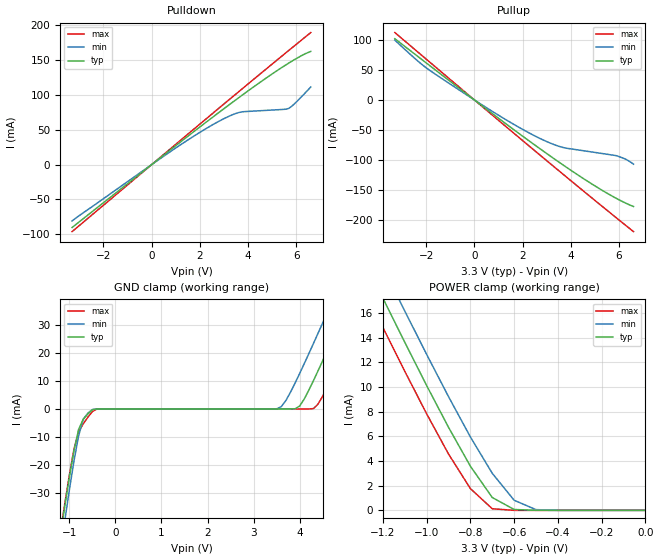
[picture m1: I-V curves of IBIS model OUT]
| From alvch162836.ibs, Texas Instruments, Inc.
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|   Model ALVCH162836_OUT
[Model]   OUT
Model_type   3-state
Polarity   Non-Inverting
Enable   Active-High
|Variable   typ   min   max
C_comp   7.0pF   NA   NA
[Voltage range]   3.3   3.0   3.6
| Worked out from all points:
|   slope of the pulldown table from 0 to 0.495 V, typ, clamps not added: 36.6 ohm
|   slope of the pullup table from 0 to 0.495 V, typ, clamps not added: 32.7 ohm
|   GND clamp passes 1 mA (typ) near -0.55 V on its own axis
|   POWER clamp passes 1 mA (typ) near -0.70 V on its own axis
[Pullup]   | Note: Vtable = Vcc - Voutput
|   Voltage   I(typ)   I(min)   I(max)
-3.3V     101.7mA    99.31mA    111.9mA
-2.3V     70.82mA    63.05mA    78mA
-1.8V     55.39mA    47.67mA    61.05mA
700mV     -21.34mA   -17.91mA   -23.7mA
2.4V      -71.8mA    -57.51mA   -80.85mA
3.1V      -91.84mA   -70.88mA   -104.2mA
3.6V      -105.8mA   -78.13mA   -120.8mA
4.9V      -140.3mA   -86.6mA    -163.6mA
5.9V      -163.8mA   -92.71mA   -196.2mA
6.3V      -171.8mA   -98.96mA   -209.1mA
6.6V      -177mA     -106.6mA   -218.7mA
[Pulldown]
|   Voltage   I(typ)   I(min)   I(max)
-3.3V     -90.25mA   -80.85mA   -96.21mA
700mV     19.09mA    16.83mA    20.42mA
1.7V      46.04mA    39.78mA    49.49mA
2.6V      69.89mA    58.61mA    75.55mA
3.2V      85.5mA     69.31mA    92.86mA
3.7V      98.3mA     75.47mA    107.2mA
5.5V      141.7mA    79.34mA    158.6mA
5.7V      146mA      80.98mA    164.3mA
6V        152.3mA    89.88mA    172.7mA
6.6V      162.5mA    111.4mA    189.6mA
[POWER_Clamp]   | Note: Vtable = Vcc - Voutput
|   Voltage   I(typ)   I(min)   I(max)
-3.3V     95.82mA    98.2mA     93.52mA
-1.3V     20.85mA    23.37mA    18.46mA
-1.2V     17.22mA    19.76mA    14.85mA
-1.1V     13.64mA    16.18mA    11.29mA
-1V       10.13mA    12.66mA    7.835mA
-900mV    6.739mA    9.228mA    4.573mA
-800mV    3.582mA    5.956mA    1.766mA
-700mV    1.041mA    3.004mA    129uA
-600mV    70.56uA    819.7uA    1.512uA
-500mV    2.077uA    58.75uA    22.94nA
0V        990pA      903.2pA    1.08nA
[GND_Clamp]
|   Voltage   I(typ)   I(min)   I(max)
-3.3V     -303.1mA   -308.7mA   -297.8mA
-1.2V     -45.81mA   -51.34mA   -44.52mA
-1.1V     -34.74mA   -39.9mA    -33.79mA
-800mV    -7.335mA   -9.635mA   -8.16mA
-400mV    -9.992nA   -367.3nA   -984.6pA
3.5V      1.134nA    58.72uA    1.03nA
4V        1.041mA    12.66mA    1.589nA
4.3V      10.13mA    23.37mA    129.1uA
4.7V      24.5mA     38.08mA    11.29mA
5.1V      39.32mA    52.99mA    25.79mA
5.4V      50.54mA    64.25mA    36.94mA
6.6V      95.82mA    109.6mA    82.15mA
[Ramp]
| variable   typ   min   max
dV/dt_r   1.1964E+00/2.2487E-10  1.0081E+00/2.9867E-10  1.3585E+00/2.1748E-10
dV/dt_f   1.1447E+00/2.2170E-10  9.8466E-01/4.0710E-10  1.2833E+00/1.8639E-10
